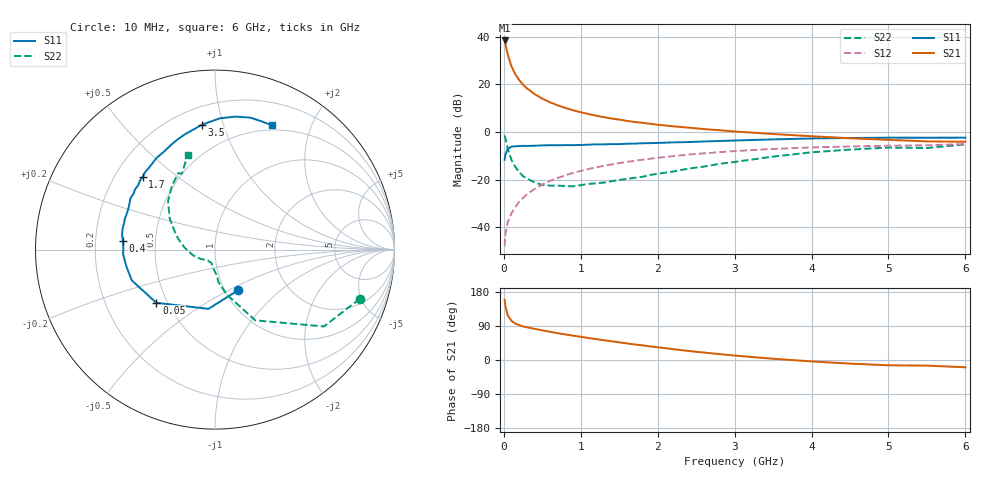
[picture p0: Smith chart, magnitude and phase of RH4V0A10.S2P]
! SIEMENS Small Signal Semiconductors
! BFR106
! Si NPN RF Bipolar Junction Transistor in SOT23
! VCE = 4 V  IC = 100 mA
! Common Emitter S-Parameters:  August  1996
# GHz  S  MA  R  50
!  f  S11  S21  S12  S22
! GHz  MAG  ANG  MAG  ANG  MAG  ANG  MAG  ANG
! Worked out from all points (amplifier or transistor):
!   36 points, 10 MHz to 6 GHz, reference 50 ohm
!   highest |S21| = 38.5 dB at 10 MHz (marker M1)
!   |S21| within 3 dB of that: start of sweep to 31.1 MHz
!   unconditionally stable (mu >= 1): 149.7 MHz to 2.559 GHz; 5.366 GHz to end of sweep
!   at 250 MHz: K = 1.07, MAG = 22.1 dB, |S12| = -27.7 dB
!   at 1.4 GHz: K = 1.07, MAG = 8.0 dB, |S12| = -13.6 dB
!   at 6 GHz: K = 1.00, MAG = 0.2 dB, |S12| = -5.0 dB
!   S11 on the Smith chart (normalised r, x): 10 MHz: 1.15, -0.56; 50 MHz: 0.44, -0.32; 400 MHz: 0.32, +0.04; 1.7 GHz: 0.32, +0.38; 3.5 GHz: 0.31, +0.85; 6 GHz: 0.45, +1.47
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0.01  0.2607 -60.6  83.97 159.2  0.004 79.2  0.852 -18.8
0.02  0.3321 -96.3  72.05 143.3  0.0071 65.4  0.7428 -35.2
0.05  0.4412 -137.8  42.85 118.0  0.0128 61.8  0.4533 -60.4
0.1  0.4941 -159.6  23.85 103.1  0.0198 65.3  0.2565 -75.6
0.15  0.5025 -169.2  16.25 96.0  0.0267 69.2  0.1835 -83.8
0.2  0.5067 -173.5  12.36 92.0  0.0344 71.8  0.1437 -86.2
0.25  0.5129 -177.4  9.887 88.6  0.0413 72.6  0.118 -91.2
0.3  0.5105 180.0  8.281 86.3  0.049 73.6  0.1064 -94.7
0.4  0.515 174.7  6.27 82.2  0.064 74.2  0.0872 -100.5
0.5  0.5241 171.0  5.033 78.2  0.079 73.8  0.0771 -105.2
0.6  0.5283 167.2  4.221 74.4  0.0941 72.8  0.0748 -109.6
0.7  0.5273 163.9  3.646 70.7  0.1086 72.1  0.075 -114.9
0.9  0.5305 157.8  2.866 64.3  0.1382 69.3  0.0724 -124.4
1.1  0.5432 151.1  2.39 58.1  0.167 66.5  0.0812 -133.0
1.4  0.558 142.7  1.923 49.5  0.2089 61.9  0.0927 -145.3
1.7  0.5715 134.9  1.627 41.0  0.2488 57.3  0.1091 -158.5
2.2  0.6061 122.4  1.319 28.7  0.3117 49.3  0.1478 -176.3
2.8  0.6482 108.8  1.093 15.7  0.3776 39.7  0.2142 163.5
3.5  0.7002 95.8  0.908 3.3  0.4419 28.9  0.305 145.7
4.5  0.7498 81.2  0.74 -9.5  0.4971 14.3  0.4275 124.3
5.5  0.7603 69.2  0.636 -14.8  0.5261 4.9  0.4617 113.5
6  0.7614 65.3  0.625 -19.2  0.5598 -2.1  0.5494 106.1
